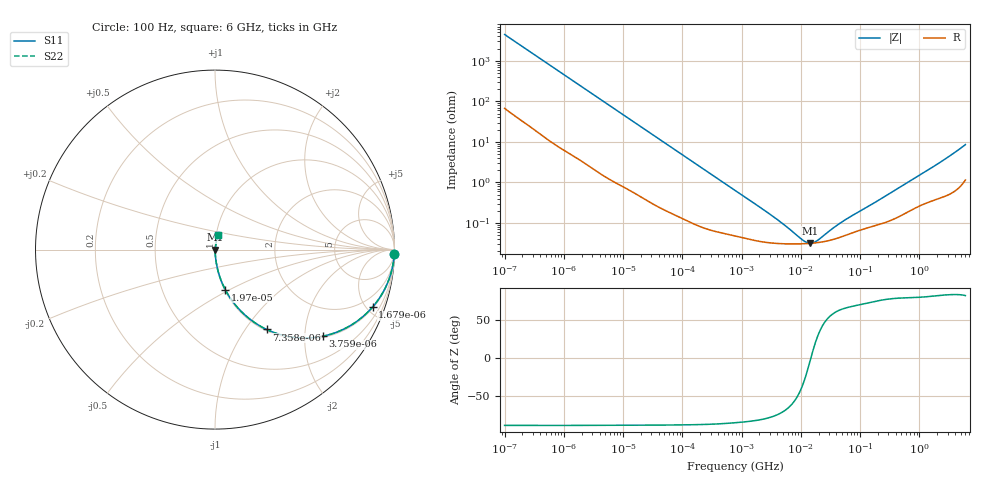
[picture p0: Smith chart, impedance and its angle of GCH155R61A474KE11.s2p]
!Murata Part Number: GCH155R61A474KE11
!These Parameters are Measured in Series Mode Connection
!Data Generated on Mar 13, 2026
!  o--ll--o
!Port1  Port2
!  o------o
!Operation Temp=25[degC], DC Bias Voltage=0[V]
!Freq. Start=100[Hz] Stop=6[GHz] 401[Steps]
# Hz S RI R 50
!Freq.(Hz) S11(Real) S11(Imag) S21(Real) S21(Imag) S12(Real) S12(Imag) S22(Real) S22(Imag)
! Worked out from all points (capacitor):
!   401 points, 100 Hz to 6 GHz, reference 50 ohm
!   read as one part in series: C = 355 nF near 109 Hz
!   lowest |Z| = 31.5 mohm at 14.22 MHz (marker M1)
!   series resonance near 14.8 MHz, so ESL is about 330 pH
!   S11 on the Smith chart (normalised r, x): 100 Hz: 2, -89; 1.679 kHz: 1.08, -5.45; 3.759 kHz: 1.04, -2.45; 7.358 kHz: 1.02, -1.26; 19.7 kHz: 1.01, -0.48; 6 GHz: 1.02, +0.17
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100  0.9992 -0.0224  0.000838 0.0224  0.000838 0.0224  0.9992 -0.0224
501  0.9865 -0.109  0.0135 0.109  0.0135 0.109  0.9865 -0.109
1026  0.9491 -0.2131  0.0509 0.2131  0.0509 0.2131  0.9491 -0.2131
1679  0.8778 -0.3204  0.1222 0.3204  0.1222 0.3204  0.8778 -0.3204
2008  0.8353 -0.3637  0.1647 0.3637  0.1647 0.3637  0.8353 -0.3637
3759  0.5991 -0.4828  0.4009 0.4828  0.4009 0.4828  0.5991 -0.4828
5143  0.4474 -0.4898  0.5526 0.4898  0.5526 0.4898  0.4474 -0.4898
7358  0.2871 -0.4446  0.7129 0.4446  0.7129 0.4446  0.2871 -0.4446
11514  0.1448 -0.3433  0.8552 0.3433  0.8552 0.3433  0.1448 -0.3433
19704  0.0572 -0.2231  0.9428 0.2231  0.9428 0.2231  0.0572 -0.2231
40335  0.0158 -0.1149  0.9842 0.1149  0.9842 0.1149  0.0158 -0.1149
129199  0.00244 -0.0369  0.9976 0.0369  0.9976 0.0369  0.00244 -0.0369
774597  0.00052 -0.00633  0.9995 0.00633  0.9995 0.00633  0.00052 -0.00633
3712478  0.000316 -0.00128  0.9997 0.00128  0.9997 0.00128  0.000316 -0.00128
1.087309e7  0.000307 -0.000214  0.9997 0.000214  0.9997 0.000214  0.000307 -0.000214
1.422411e7  0.000314 -2.72e-05  0.9997 2.72e-05  0.9997 2.72e-05  0.000314 -2.72e-05
1.555665e7  0.000317 3.37e-05  0.9997 -3.37e-05  0.9997 -3.37e-05  0.000317 3.37e-05
1.946e7  0.000329 0.000187  0.9997 -0.000187  0.9997 -0.000187  0.000329 0.000187
5.449875e7  0.000485 0.00106  0.9995 -0.00106  0.9995 -0.00106  0.000485 0.00106
3.124326e8  0.00114 0.00517  0.9989 -0.00517  0.9989 -0.00517  0.00114 0.00517
1.95892e9  0.00454 0.027  0.9955 -0.027  0.9955 -0.027  0.00454 0.027
6e9  0.0183 0.0824  0.9817 -0.0824  0.9817 -0.0824  0.0183 0.0824
